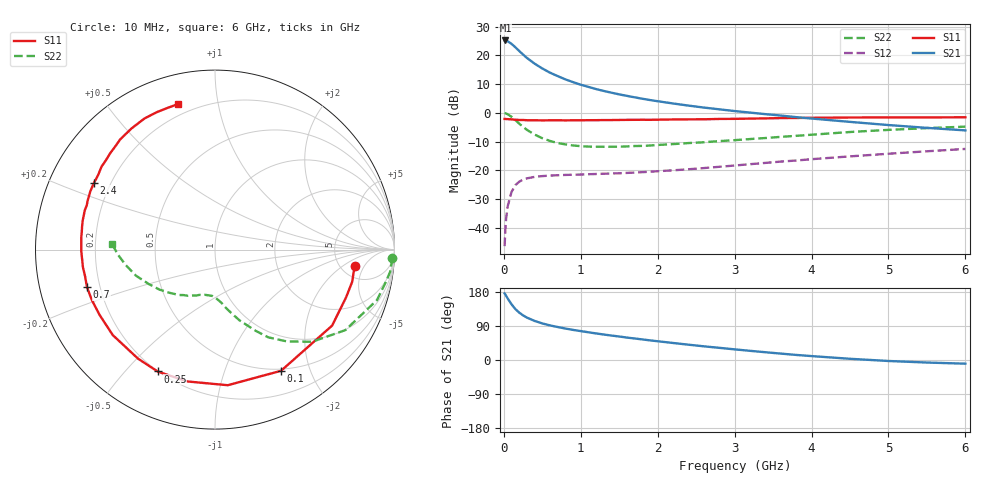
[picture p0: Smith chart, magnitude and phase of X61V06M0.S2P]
! SIEMENS Small Signal Semiconductors
! BFP193W
! Si NPN RF Bipolar Junction Transistor in SOT343
! VCE = 1 V  IC = 6 mA
! Common Emitter S-Parameters:  April 1994
# GHz  S  MA  R  50
!  f  S11  S21  S12  S22
! GHz  MAG  ANG  MAG  ANG  MAG  ANG  MAG  ANG
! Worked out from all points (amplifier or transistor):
!   40 points, 10 MHz to 6 GHz, reference 50 ohm
!   highest |S21| = 25.2 dB at 20 MHz (marker M1)
!   |S21| within 3 dB of that: start of sweep to 174.1 MHz
!   unconditionally stable (mu >= 1): 1.496 GHz to end of sweep
!   at 200 MHz: K = 0.16, MSG = 22.7 dB, |S12| = -24.0 dB
!   at 1.5 GHz: K = 1.00, MAG = 13.4 dB, |S12| = -21.0 dB
!   at 6 GHz: K = 1.01, MAG = 2.8 dB, |S12| = -12.6 dB
!   S11 on the Smith chart (normalised r, x): 10 MHz: 6.75, -3.15; 100 MHz: 0.48, -1.58; 250 MHz: 0.20, -0.62; 700 MHz: 0.15, -0.14; 2.4 GHz: 0.14, +0.25; 6 GHz: 0.14, +0.77
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0.01  0.7836 -6.6  18.13 175.6  0.0048 88.9  0.9893 -2.7
0.02  0.785 -13.3  18.14 172.8  0.0097 81.0  0.9837 -7.2
0.03  0.7773 -20.0  18.03 169.3  0.0147 80.4  0.9698 -10.5
0.05  0.7778 -33.0  17.57 162.3  0.0237 74.2  0.9454 -17.3
0.1  0.769 -61.4  15.83 147.0  0.0422 60.5  0.8537 -31.7
0.15  0.7589 -84.6  13.8 134.4  0.0553 49.8  0.7461 -43.5
0.2  0.7509 -102.0  11.88 125.0  0.0634 42.6  0.649 -52.0
0.25  0.7505 -115.2  10.33 117.8  0.0691 36.8  0.5723 -58.7
0.3  0.7437 -125.2  9.011 111.9  0.0726 32.9  0.5061 -63.4
0.4  0.7424 -140.1  7.162 103.1  0.0769 27.7  0.4183 -70.8
0.5  0.7389 -150.4  5.903 96.5  0.0794 24.9  0.3621 -75.9
0.6  0.7414 -157.5  4.994 91.3  0.0811 23.1  0.3243 -80.1
0.7  0.7435 -163.6  4.35 87.0  0.0822 22.4  0.2986 -83.1
0.9  0.7424 -172.4  3.418 79.4  0.0839 22.0  0.2707 -88.8
1.1  0.7449 -179.2  2.825 73.1  0.0856 22.6  0.2585 -93.5
1.6  0.7547 167.6  1.973 59.2  0.0902 26.6  0.2605 -104.0
2.2  0.7667 155.0  1.454 44.9  0.1001 32.0  0.2858 -116.4
2.4  0.7699 151.2  1.336 40.4  0.1044 33.7  0.298 -120.2
3.2  0.7937 137.2  1.01 24.2  0.1279 38.0  0.3498 -136.5
4.5  0.8294 118.3  0.696 3.2  0.1749 37.3  0.4641 -161.8
5.5  0.8324 108.8  0.548 -6.7  0.2145 33.3  0.5425 -177.2
6  0.8366 104.3  0.495 -9.7  0.2356 31.1  0.5755 176.7
